(* Logix 5000 AddOnInstructionDefinition export AMCI_5034_PTO_AM_Registration; software revision 37.00 *)

TYPE AMCI_5034_PTO_AM_Input_Data :
STRUCT
   ConnectionFaulted : DINT;
   MovingCW : BOOL;
   MovingCCW : BOOL;
   InHoldState : BOOL;
   Stopped : BOOL;
   AtHome : BOOL;
   Accelerating : BOOL;
   Decelerating : BOOL;
   MoveComplete : BOOL;
   HomeInvalid : BOOL;
   InvalidProfile : BOOL;
   PositionInvalid : BOOL;
   InputError : BOOL;
   CommandError : BOOL;
   ConfigurationError : BOOL;
   ModuleOK : BOOL;
   GeneralPurposeOutputStatus : BOOL;
   Input1Active : BOOL;
   Input2Active : BOOL;
   Input3Active : BOOL;
   Input4Active : BOOL;
   bit_20_reserved : BOOL;
   bit_21_reserved : BOOL;
   bit_22_reserved : BOOL;
   EncoderFollowerMode : BOOL;
   BlendMoveRunning : BOOL;
   BlendMoveAcknowledge : BOOL;
   MinimumRegistrationProgrammed : BOOL;
   EncoderMotionDirection : BOOL;
   MultipleInputsWithSameFunction : BOOL;
   FSCExceedsNumberOfDataBits : BOOL;
   AbsoluteEncoderSetupError : BOOL;
   bit_31_reserved : BOOL;
   CurrentPosition : DINT;
   EncoderPosition : DINT;
   CapturedPosition : DINT;
END_STRUCT
END_TYPE

TYPE AMCI_5034_PTO_AM_Output_Data :
STRUCT
   Command_Word : DINT;
   TargetPosition : DINT;
   TargetVelocity : UDINT;
   Acceleration : DINT;
   Deceleration : DINT;
END_STRUCT
END_TYPE

ADD_ON_INSTRUCTION AMCI_5034_PTO_AM_Registration   (* revision 1.0, vendor AMCI, ExecuteEnableInFalse *)
// AMCI Registration Move
// Revision note:
// 10/1/2025 Initial release of AOI.  Making the rung false will stop the registration move
// Help:
// Performs CW or CCW Registration Moves
// AXIS INPUT DATA:  Input data from the AMCI 5034-PTO-AM.   Uses the AMCI_5034_PTO_Input_Data User Defined Data Type.
// AXIS OUTPUT DATA; Output data from the AOI to the AMCI 5034-PTO-AM.    Uses the AMCI_5034_PTO_Output_Data User Defined Data Type.
// DIRECTION: 0 for Positve CW  or 1 for Negative CCW
// REGISTRATION_DISTANCE: Distance to move after the Registration Input has become active.
// TARGETVELOCITY: Speed of move in units of steps / sec
// ACCELERATION: Acceleration Rate in units of steps / sec / ms
// DECELERATION:  Deceleration Rate in units of steps / sec / ms
// EN (Enable) Set when rung is true, Reset when rung is false
// DN (Done) Set when command is sent to the motion device.  Reset when the rung is false.
// ER (Error) Set when a command, input. or configuration error.  Reset when the rung is false.
// IP (In Process) Set when motion is occurring.   Reset when motion stops or the rung goes false.
VAR_IN_OUT
   Axis_Input_Data : AMCI_5034_PTO_AM_Input_Data; {required}
   Axis_Output_Data : AMCI_5034_PTO_AM_Output_Data; {required}
END_VAR
VAR_INPUT
   Direction_0_PositiveCW_1_NegativeCCW : BOOL; {required}   // 0=jog CW 1=jog CCW
   _0_normal_1_S_Curve_Acceleration : BOOL;
   _0_Triangular_1_Trapezoidal_S_Curve : BOOL;
   Registration_Distance : DINT; {required}
   Programmed_Speed : DINT; {required}
   Acceleration : DINT; {required}
   Deceleration : INT; {required}
END_VAR
VAR_OUTPUT
   EN : BOOL; {visible}   // set when rung with AOI is true
   DN : BOOL; {access Read Only, visible}   // set when move was succesfully initiated
   ER : BOOL; {visible}
   IP : BOOL; {visible}   // set when motion occurring
END_VAR
VAR
   command_data_block : DINT[5];
        [0]   // Command Word
        [1]   // Target Positon
        [2]   // Programmed Speed
        [3]   // Acceleration
        [4]   // Deceleration
   motion_occurring : BOOL; {access None}
   Internal_Enable : BOOL; {access None}   // set when driver ready to receive motion command
END_VAR

ROUTINE EnableInFalse   (* ladder *)
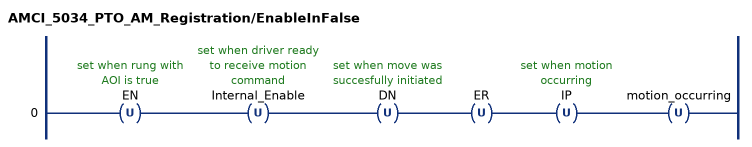
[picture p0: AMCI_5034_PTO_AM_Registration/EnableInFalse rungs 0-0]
   0: OTU(EN)OTU(Internal_Enable)OTU(DN)OTU(ER)OTU(IP)OTU(motion_occurring);
END_ROUTINE

ROUTINE Logic   (* ladder *)
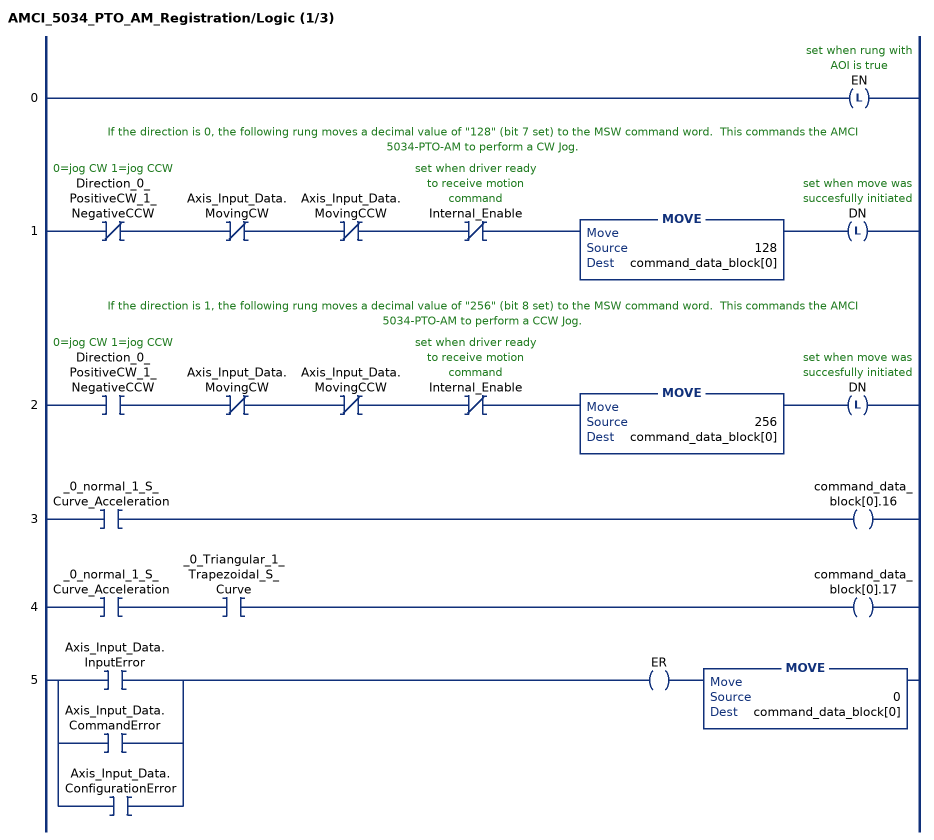
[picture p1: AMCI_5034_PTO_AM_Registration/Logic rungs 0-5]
   0: OTL(EN);
   // If the direction is 0, the following rung moves a decimal value of "128" (bit 7 set) to the MSW command word.  This commands the AMCI 5034-PTO-AM to perform a CW Jog.
   1: XIO(Direction_0_PositiveCW_1_NegativeCCW)XIO(Axis_Input_Data.MovingCW)XIO(Axis_Input_Data.MovingCCW)XIO(Internal_Enable)MOVE(128,command_data_block[0])OTL(DN);
   // If the direction is 1, the following rung moves a decimal value of "256" (bit 8 set) to the MSW command word.  This commands the AMCI 5034-PTO-AM to perform a CCW Jog.
   2: XIC(Direction_0_PositiveCW_1_NegativeCCW)XIO(Axis_Input_Data.MovingCW)XIO(Axis_Input_Data.MovingCCW)XIO(Internal_Enable)MOVE(256,command_data_block[0])OTL(DN);
   3: XIC(_0_normal_1_S_Curve_Acceleration)OTE(command_data_block[0].16);
   4: XIC(_0_normal_1_S_Curve_Acceleration)XIC(_0_Triangular_1_Trapezoidal_S_Curve)OTE(command_data_block[0].17);
   5: [XIC(Axis_Input_Data.InputError) ,XIC(Axis_Input_Data.CommandError) ,XIC(Axis_Input_Data.ConfigurationError) ]OTE(ER)MOVE(0,command_data_block[0]);
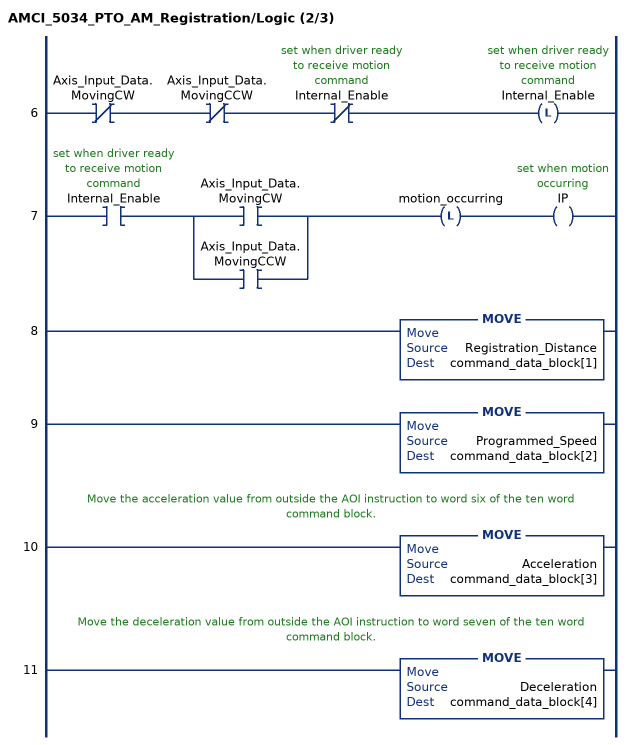
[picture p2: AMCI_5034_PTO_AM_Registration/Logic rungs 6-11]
   6: XIO(Axis_Input_Data.MovingCW)XIO(Axis_Input_Data.MovingCCW)XIO(Internal_Enable)OTL(Internal_Enable);
   7: XIC(Internal_Enable)[XIC(Axis_Input_Data.MovingCW) ,XIC(Axis_Input_Data.MovingCCW) ]OTL(motion_occurring)OTE(IP);
   8: MOVE(Registration_Distance,command_data_block[1]);
   9: MOVE(Programmed_Speed,command_data_block[2]);
   // Move the acceleration value from outside the AOI instruction to word six of the ten word command block.
   10: MOVE(Acceleration,command_data_block[3]);
   // Move the deceleration value from outside the AOI instruction to word seven of the ten word command block.
   11: MOVE(Deceleration,command_data_block[4]);
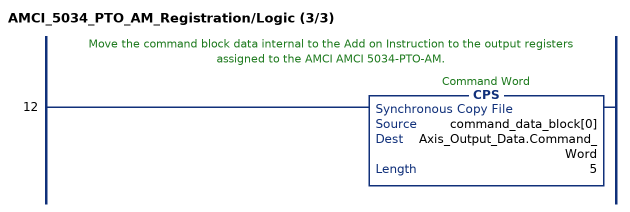
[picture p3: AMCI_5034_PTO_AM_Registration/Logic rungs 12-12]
   // Move the command block data internal to the Add on Instruction to the output registers assigned to the AMCI AMCI 5034-PTO-AM.
   12: CPS(command_data_block[0],Axis_Output_Data.Command_Word,5);
END_ROUTINE
END_ADD_ON_INSTRUCTION
